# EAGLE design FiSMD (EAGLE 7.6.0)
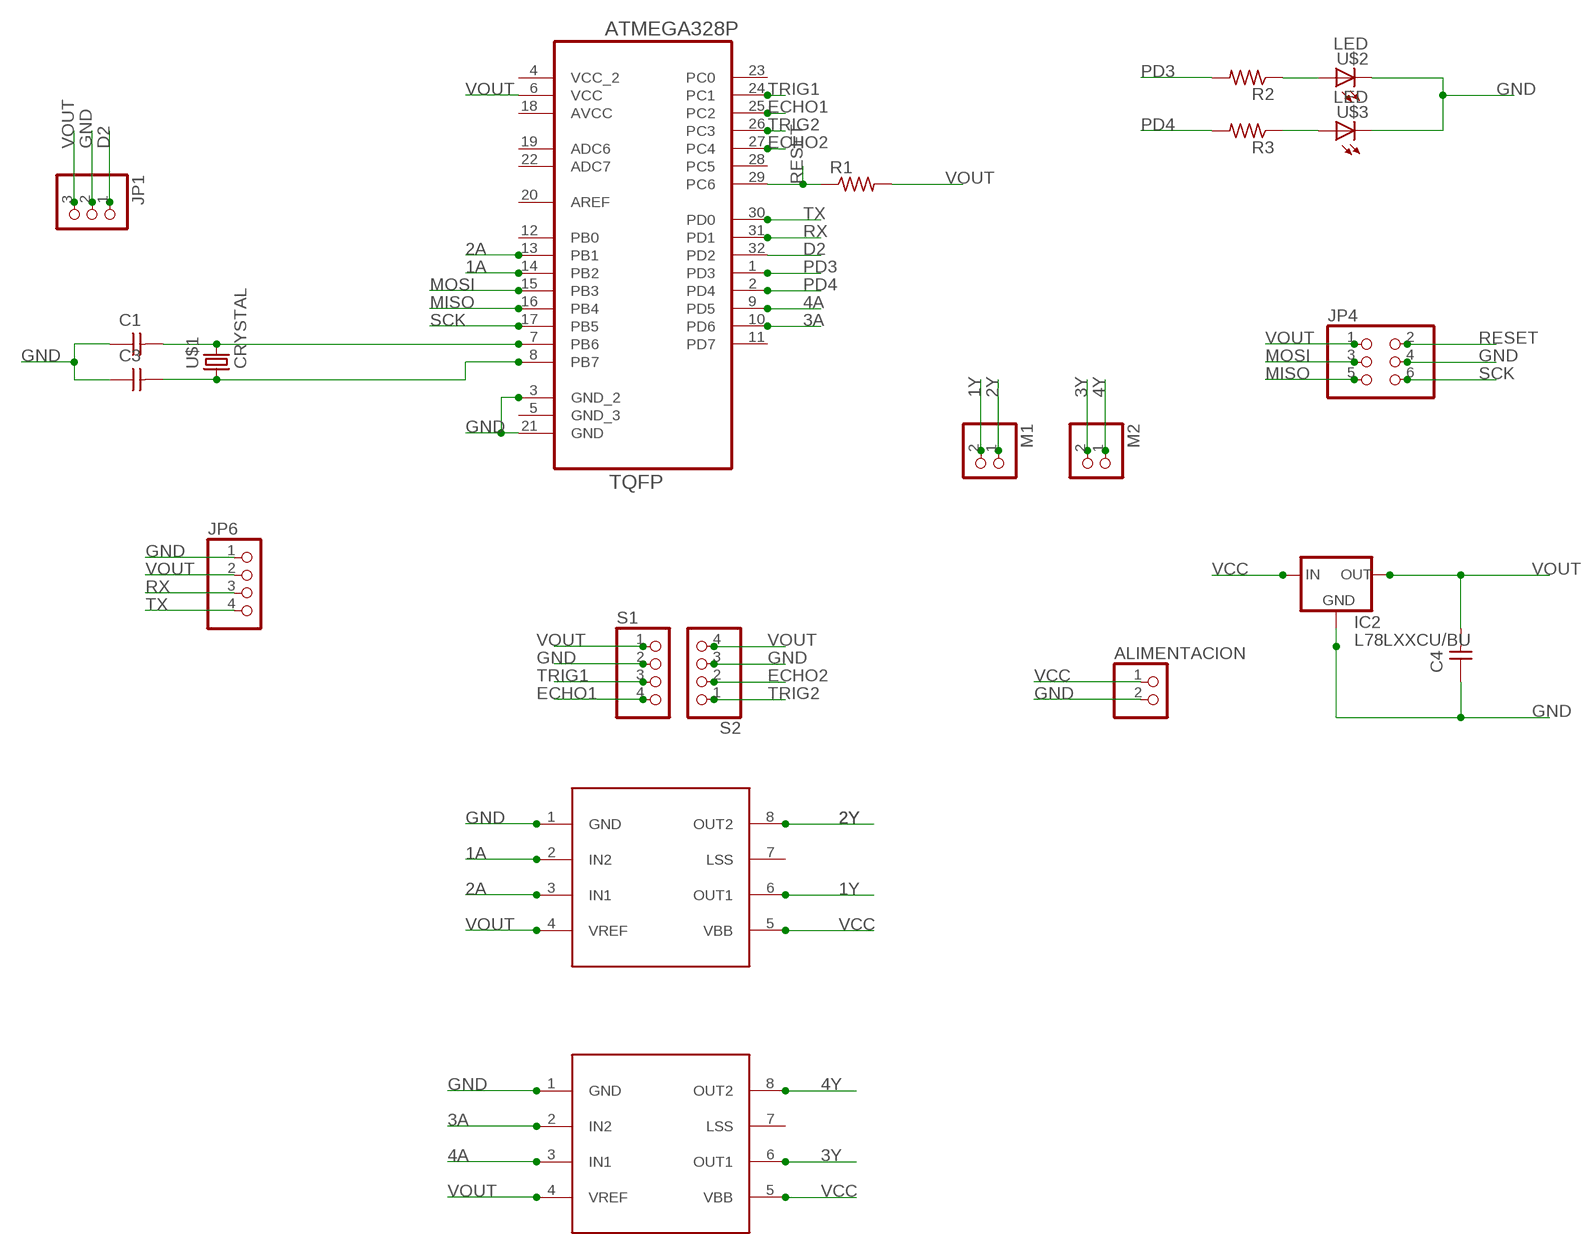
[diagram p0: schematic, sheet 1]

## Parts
ALIMENTACION  PINHD-1X2  [1X02]
C1  CAP-UNPOLARIZED  [C1206]
C3  CAP-UNPOLARIZED  [C1206]
C4  CAP-UNPOLARIZED  [C1206]
D1  A4953-H-BRIDGE-MOTOR-DRIVER  [SOIC8]
D2  A4953-H-BRIDGE-MOTOR-DRIVER  [SOIC8]
IC2  L78LXXCU/BU  [SOT89]
JP1  PINHD-1X3  [1X03]
JP4  PINHD-2X3  [2X03]
JP6  PINHD-1X4  [1X04]
M1  PINHD-1X2  [1X02]
M2  PINHD-1X2  [1X02]
R1  RES-US1206  [R1206]
R2  RES-US1206  [R1206]
R3  RES-US1206  [R1206]
S1  PINHD-1X4  [1X04]
S2  PINHD-1X4  [1X04]
U1  ATMEGA328P-AU  [QFP80P900X900X120-32N]
U$1  CRYSTAL  [2-SMD-5X3MM]
U$2  LED  [LED1206]
U$3  LED  [LED1206]

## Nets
1A: D1.2(IN2) U1.14(PB2)
1Y: D1.6(OUT1) M1.2
2A: D1.3(IN1) U1.13(PB1)
2Y: D1.8(OUT2) M1.1
3A: D2.2(IN2) U1.10(PD6)
3Y: D2.6(OUT1) M2.2
4A: D2.3(IN1) U1.9(PD5)
4Y: D2.8(OUT2) M2.1
D2: JP1.1 U1.32(PD2)
ECHO1: S1.4 U1.25(PC2)
ECHO2: S2.2 U1.27(PC4)
GND: ALIMENTACION.2 C1.1 C3.1 C4.1 D1.1(GND) D2.1(GND) IC2.2(GND) IC2.4(GND1) JP1.2 JP4.4 JP6.1 S1.2 S2.3 U1.3(GND_2) U1.21(GND) U$2.2(C) U$3.2(C)
MISO: JP4.5 U1.16(PB4)
MOSI: JP4.3 U1.15(PB3)
N$1: R2.1 U$2.1(A)
N$2: C1.2 U1.7(PB6) U$1.P$2
N$3: C3.2 U1.8(PB7) U$1.P$1
N$5: R3.1 U$3.1(A)
PD3: R2.2 U1.1(PD3)
PD4: R3.2 U1.2(PD4)
RESET: JP4.2 R1.1 U1.29(PC6)
RX: JP6.3 U1.31(PD1)
SCK: JP4.6 U1.17(PB5)
TRIG1: S1.3 U1.24(PC1)
TRIG2: S2.1 U1.26(PC3)
TX: JP6.4 U1.30(PD0)
VCC: ALIMENTACION.1 D1.5(VBB) D2.5(VBB) IC2.3(IN)
VOUT: C4.2 D1.4(VREF) D2.4(VREF) IC2.1(OUT) JP1.3 JP4.1 JP6.2 R1.2 S1.1 S2.4 U1.6(VCC)
Unconnected: D1.7(LSS) D2.7(LSS) U1.5(GND_3) U1.11(PD7) U1.12(PB0) U1.19(ADC6) U1.20(AREF) U1.22(ADC7) U1.23(PC0) U1.28(PC5)

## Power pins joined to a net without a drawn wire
AVCC: U1.18(AVCC)
VCC_2: U1.4(VCC_2)

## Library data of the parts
ALIMENTACION M1 M2 = pinhead:PINHD-1X2: PIN HEADER
C1 C3 C4 = fab:CAP-UNPOLARIZED
D1 D2 = fab:A4953-H-BRIDGE-MOTOR-DRIVER
IC2 = v-reg-2:L78LXXCU/BU: VOLTAGE REGULATOR
JP1 = pinhead:PINHD-1X3: PIN HEADER
JP4 = pinhead:PINHD-2X3: PIN HEADER
JP6 S1 S2 = pinhead:PINHD-1X4: PIN HEADER
R1-R3 = fab:RES-US: Resistor (US Symbol)
U1 = Ava:ATMEGA328P-AU; DESCRIPTION: 8-bit Microcontroller with In-System Programmable Flash; MPN: ATMEGA328P-AU; OC_FARNELL: 1715486; OC_NEWARK: 14R4631; PACKAGE: TQFP-32; SUPPLIER: Atmel
U$1 = fab:CRYSTAL
U$2 U$3 = fab:LED: LED

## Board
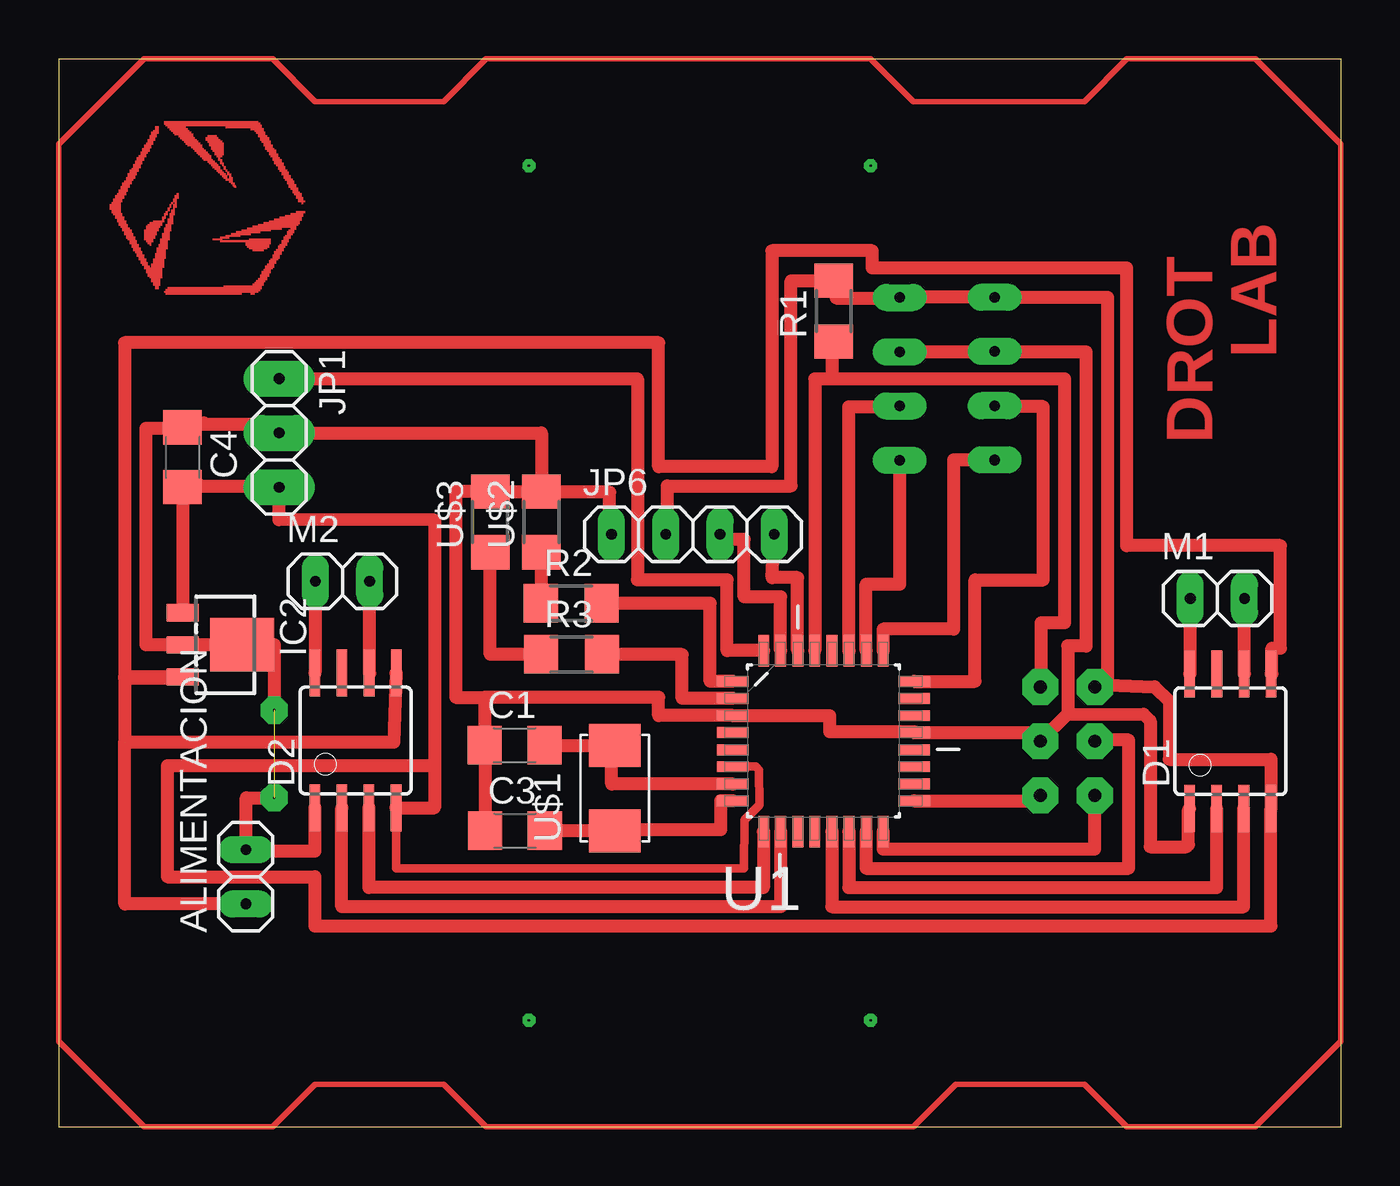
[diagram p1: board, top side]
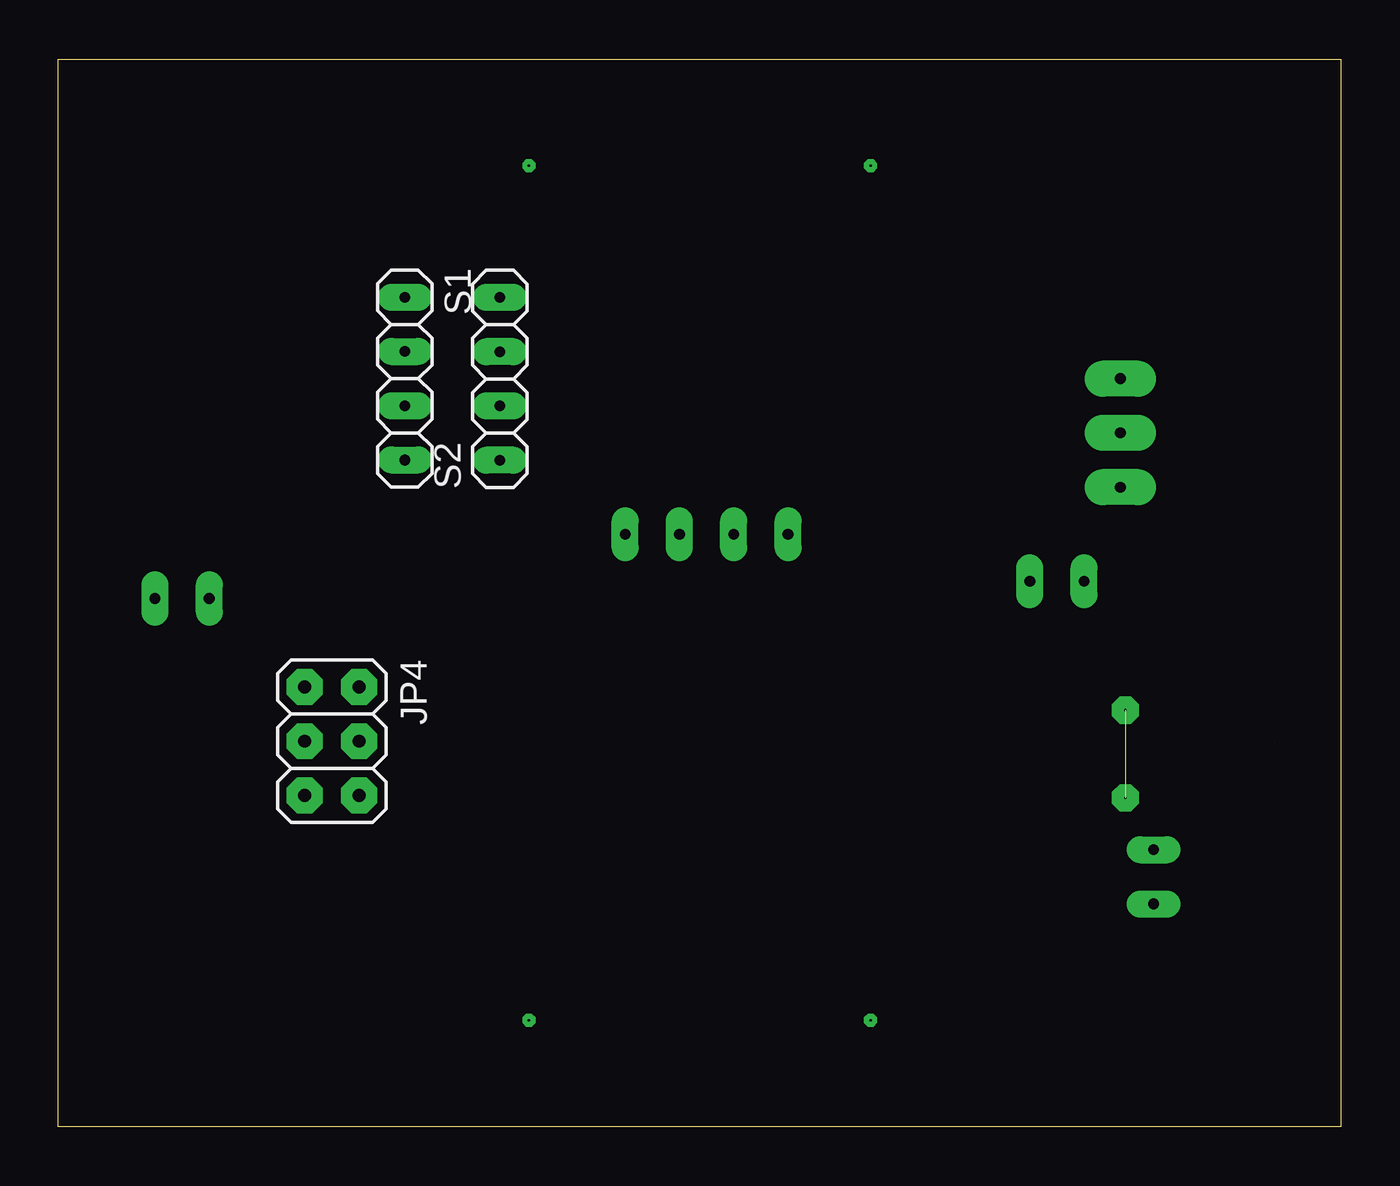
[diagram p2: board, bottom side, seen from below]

Size 60.03 x 49.97 mm. Coordinates in mm from the lower left corner, seen from the top.
Outline: 0,0 60.03,0 60.03,49.97 0,49.97 0,0
Copper layers (1*16): Top 0.035mm / dielectric 1.5mm / Bottom 0.035mm
Design rules "default": minimum track width 10mil, minimum drill 24mil, track to track 8mil, track to pad 8mil, pad to pad 8mil, via to via 8mil, smd to smd 8mil, copper to edge 40mil, drill to drill 8mil, minimum pad ring 10mil, minimum via ring 8mil, stop-mask expansion 4mil, vias tented up to drill 0mil, thermal gap 10mil

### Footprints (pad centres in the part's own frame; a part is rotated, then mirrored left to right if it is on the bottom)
1X02 = drill 0.5 pad 1.27 long: 1 -1.27,0; 2 1.27,0
C1206 = smd 1.6 x 1.8: 1 -1.4,0; 2 1.4,0
SOIC8 = smd 0.5 x 2.2: 1 -1.905,-3.154; 2 -0.645,-3.154; 3 0.625,-3.154; 4 1.895,-3.154; 5 1.905,3.154; 6 0.635,3.154; 7 -0.635,3.154; 8 -1.905,3.154
SOT89 = smd 0.8 x 1.5: 1 -1.5,-1.75; 2 0,-1.75; 3 1.5,-1.75 | smd 2.5 x 3: 4 0,1.05
1X03 = drill 0.5 pad 1.676 long: 1 -2.54,0; 2 0,0; 3 2.54,0
2X03 = drill 0.6 pad 1.676 octagon: 1 -2.54,-1.27; 2 -2.54,1.27; 3 0,-1.27; 4 0,1.27; 5 2.54,-1.27; 6 2.54,1.27
1X04 = drill 0.5 pad 1.27 long: 1 -3.81,0; 2 -1.27,0; 3 1.27,0; 4 3.81,0
R1206 = smd 1.6 x 1.803: 1 -1.422,0; 2 1.422,0
QFP80P900X900X120-32N = smd 1.473 x 0.508: 1 -4.242,2.794; 2 -4.242,2.007; 3 -4.242,1.194; 4 -4.242,0.406; 5 -4.242,-0.406; 6 -4.242,-1.194; 7 -4.242,-2.007; 8 -4.242,-2.794; 17 4.242,-2.794; 18 4.242,-2.007; 19 4.242,-1.194; 20 4.242,-0.406; 21 4.242,0.406; 22 4.242,1.194; 23 4.242,2.007; 24 4.242,2.794 | smd 0.508 x 1.473: 9 -2.794,-4.242; 10 -2.007,-4.242; 11 -1.194,-4.242; 12 -0.406,-4.242; 13 0.406,-4.242; 14 1.194,-4.242; 15 2.007,-4.242; 16 2.794,-4.242; 25 2.794,4.242; 26 2.007,4.242; 27 1.194,4.242; 28 0.406,4.242; 29 -0.406,4.242; 30 -1.194,4.242; 31 -2.007,4.242; 32 -2.794,4.242
2-SMD-5X3MM = smd 2 x 2.4: P$1 -2,0; P$2 2,0
LED1206 = smd 1.6 x 1.803: 1 -1.422,0; 2 1.422,0

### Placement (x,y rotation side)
ALIMENTACION  8.75,11.71 90 top
C1  21.33,17.87 0 top
C3  21.35,13.87 0 top
C4  5.79,31.35 270 top
D1  54.84,18.06 0 top
D2  13.89,18.09 0 top
IC2  7.54,22.57 270 top
JP1  10.31,32.49 270 top
JP4  47.22,18.06 270 bottom
JP6  29.68,27.74 0 top
M1  54.23,24.74 0 top
M2  13.28,25.54 0 top
R1  36.27,38.19 90 top
R2  23.98,24.52 0 top
R3  24,22.12 0 top
S1  43.81,35.03 270 bottom
S2  39.36,35.02 90 bottom
U1  35.79,18.06 0 top
U$1  26.02,15.86 90 top
U$2  22.59,28.32 90 top
U$3  20.19,28.32 90 top

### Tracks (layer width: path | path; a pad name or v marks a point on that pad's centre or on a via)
1A
  Top 0.61: U1.14 36.98,11.21 54.2,11.21 D1.2
1Y
  Top 0.61: D1.6 55.5,21.21 M1.2
2A
  Top 0.61: U1.13 36.18,13.82 36.18,10.31 55.47,10.31 D1.3
2Y
  Top 0.61: D1.8 52.96,21.21 M1.1
3A
  Top 0.61: U1.10 33.78,10.31 13.24,10.31 D2.2
3Y
  Top 0.61: D2.6 14.55,21.24 M2.2
4A
  Top 0.61: U1.9 32.98,13.82 32.98,11.21 14.52,11.21 D2.3
4Y
  Top 0.61: D2.8 12.01,21.34 M2.1
D2
  Top 0.61: U1.32 31.28,22.3 31.28,25.61 27.08,25.61 27.08,35.03 JP1.1
ECHO1
  Top 0.61: S1.4 41.88,31.22 41.88,23.31 38.58,23.31 U1.25
ECHO2
  Top 0.61: U1.27 36.98,33.71 39.86,33.71 S2.2
GND  (1 unrouted)
  Top 0.61: C3.1 19.95,17.87 C1.1 19.93,20.11 | U$2.2 U$3.2 18.58,29.74 18.58,20.11 19.93,20.11 | 47.23,19.33 45.95,18.08 JP4.4 45.95,18.47 U1.21 40.03,18.51 36.08,18.51 36.08,19.25 U1.3 28.08,19.25 28.08,20.11 19.93,20.11 | 47.23,19.33 50.78,19.32 51.08,19.01 51.08,13.11 52.78,13.11 52.88,13.21 52.88,14.85 D1.1 | S1.2 S2.3 48.08,36.29 48.08,22.51 47.23,22.52 47.23,19.33 | JP6.1 25.78,28.04 25.78,29.71 22.59,29.71 U$2.2 | U$2.2 22.59,32.49 JP1.2 10.31,32.91 6.48,32.91 6.78,32.95 C4.1 6.19,32.71 4.08,32.71 4.08,22.57 IC2.4 | IC2.4 IC2.2 | 8.18,12.91 8.78,12.91 | 8.78,12.91 8.85,13.01 ALIMENTACION.2 | D2.1 11.98,12.91 8.78,12.91 | 8.78,12.91 8.78,15.41 10.08,15.41 | IC2.4 10.08,22.57 10.08,19.51
MISO
  Top 0.61: U1.16 38.58,13.01 48.49,13.01 JP4.5
MOSI
  Top 0.61: U1.15 37.78,13.82 37.78,12.11 50.08,12.11 50.08,18.11 48.49,18.11 JP4.3
N$1
  Top 0.61: R2.1 22.59,24.52 U$2.1
N$2
  Top 0.61: C1.2 U$1.P$2 | U1.7 25.88,16.05 25.88,18.31 26.02,18.31 U$1.P$2 | U$1.P$2
N$3
  Top 0.61: C3.2 23.75,13.86 U$1.P$1 27.02,13.91 30.98,13.91 30.98,15.27 U1.8
N$5
  Top 0.61: R3.1 20.19,22.12 U$3.1
N$7  (via drill 0.1 pad 1.27)
  other vias: 10.08,19.51
N$8  (via drill 0.1 pad 1.27)
  other vias: 10.08,15.41
N$9  (via drill 0.1 pad 0.61)
  other vias: 22,45
N$10  (via drill 0.1 pad 0.61)
  other vias: 38,45
N$11  (via drill 0.1 pad 0.61)
  other vias: 38,5
N$12
  Top 0.254: 0,4 4,0 10,0 12,2 18,2 20,0 40,0 42,2 48,2 50,0 56,0 60,4 60,46 56,50 50,50 48,48 40,48 38,50 20,50 18,48 12,48 10,50 4,50 0,46 0,4
N$13  (via drill 0.1 pad 0.61)
  other vias: 22,5
N$20
  Top 0.003: 7.93,41.46 7.68,41.46 7.59,41.55
PD3
  Top 0.61: U1.1 30.48,20.85 30.48,24.51 R2.2
PD4
  Top 0.61: U1.2 29.18,20.07 29.18,22.11 R3.2
RESET
  Top 0.61: JP4.2 45.98,20.6 45.98,23.61 47.08,23.61 47.08,35.01 36.18,35.01 | 36.18,35.01 35.38,35.01 U1.29 | R1.1 36.18,36.77 36.18,35.01
RX
  Top 0.61: U1.31 33.78,24.81 32.08,24.81 32.08,27.51 30.85,27.51 JP6.3
SCK
  Top 0.61: U1.17 45.7,15.27 JP4.6
TRIG1
  Top 0.61: U1.24 42.88,20.85 42.88,25.61 46.08,25.61 46.08,33.71 43.81,33.71 S1.3
TRIG2
  Top 0.61: U1.26 37.78,22.3 37.78,25.41 39.36,25.41 S2.1
TX
  Top 0.61: U1.30 34.58,22.3 34.58,25.71 33.39,25.71 JP6.4
VCC  (1 unrouted)
  Top 0.61: ALIMENTACION.1 3.09,10.44 3.09,18.01 | D2.5 15.68,18.01 3.09,18.01 | 3.09,18.01 3.08,18.01 3.08,21.01 | IC2.3 5.58,21.07 | 5.58,21.07 3.08,21.07 | 3.08,21.07 3.08,21.01 | D1.5 56.78,21.21 56.78,22.41 57.18,22.41 57.18,27.21 49.98,27.21 49.98,40.21 38.08,40.21 38.08,41.01 33.38,41.01 33.38,30.91 28.08,30.91 28.08,36.71 3.08,36.71 3.08,21.07 | 3.08,21.01 5.48,21.01 5.58,21.07
VOUT
  Top 0.406: U1.6 32.62,16.87 32.78,16.71 32.8,15.08 32.1,14.38 32.08,12.11 15.79,12.11 D2.4
  Top 0.61: JP4.1 49.08,20.7 | 49.08,20.7 51.29,20.6 51.98,19.91 51.98,17.21 56.73,17.21 D1.4 56.73,9.41 11.98,9.41 11.98,11.71 5.08,11.71 5.08,16.91 17.58,16.91 | 49.08,20.7 49.09,38.84 S1.1 39.86,38.84 S2.4 39.36,38.81 36.38,38.81 36.38,39.61 R1.2 34.28,39.61 34.28,30.01 28.48,30.01 28.48,28.04 JP6.2 | IC2.1 C4.2 6.58,30.05 6.58,30.01 10.31,30.01 JP1.3 10.31,28.43 17.58,28.41 17.58,16.91 | D2.4 17.58,14.94 17.58,16.91
(copper drawn outside any net)
  shapes: Top area x355

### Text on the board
Top: LAB | DROT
